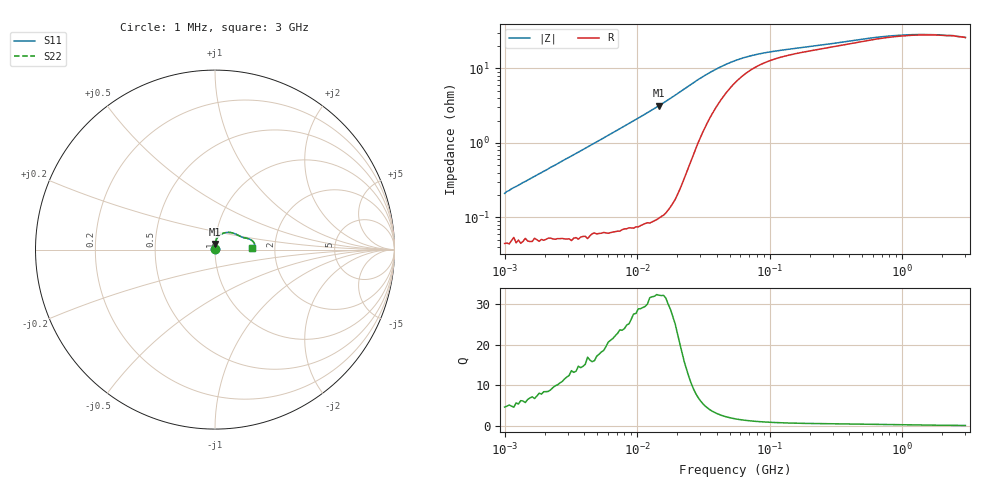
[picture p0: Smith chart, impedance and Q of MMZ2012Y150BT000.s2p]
! S-parameter Generated by TDK Corporation
! Copyright(C) 2016 TDK Corporation.
! All Rights Reserved.
! TDK P/N: MMZ2012Y150BT000 (Chip Beads)
! Property: |Z|=15¶ at 100MHz
! Size(LxWxT): 2x1.25x0.85mm, 0.079x0.049x0.033inches
! Model Type: s2p (Touchstone File Format Version 1.0)
! Frequency: DC=Yes Start=1MHz Stop=3000MHz 202points Log-sweep
! Note: This model was converted from impedance.
! Model Generated on May. 16, 2016
! Hash(MD5):
! Port Assignments:
!  1 ---@@@--- 2
! Applicable Conditions:
!  Temperature = 25 degC
!  DC Bias Current = 0 A
!  Small Signal Operation
! Terms and conditions regarding TDK Simulation Models
! (1)This simulation model is being provided solely for informational purposes. Please refer to the specifications of the products in terms of detailed characteristics of such products.
! (2)In no event shall TDK Corporation of any of its subsidiaries be liable for any loss or damage arising, directly or indirectly,
!  From any information contained in this simulation model, including, but not limited to loss or damages arising from any inaccuracies, omissions or errors in connection with such information.
! (3)Any and all copyrights on this simulation model are owned by TDK Corporation.
!  Duplication or redistribution of this simulation model without prior written permission from TDK Corporation is prohibited.
! (4)This simulation model is subject to any modification or change without any prior notice.
! (5)Neither TDK Corporation nor any of its subsidiaries shall make any warranty, express or implied,
!  Including but not limited to the correctness, implied warranties of merchantability and fitness for a particular purpose with respect to this simulation models.
! (6)The use of this simulation model shall be deemed to have consented to the terms and conditions hereof.
# MHz S MA R 50
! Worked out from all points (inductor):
!   201 points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, 1 MHz to 3 GHz, reference 50 ohm
!   read as one part in series: L = 33.4 nH near 1.041 MHz
!   highest Q = 32.1 at 14.62 MHz (marker M1), where L = 34.4 nH
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1  0.002106 77.6  0.9996 -0.1  0.9996 -0.1  0.002106 77.6
1.040844  0.002237 78.2  0.9995 -0.1  0.9995 -0.1  0.002237 78.2
1.083356  0.0023 78.8  0.9996 -0.1  0.9996 -0.1  0.0023 78.8
1.127605  0.002426 78.2  0.9995 -0.1  0.9995 -0.1  0.002426 78.2
2.055611  0.004312 83.0  0.9995 -0.2  0.9995 -0.2  0.004312 83.0
2.226959  0.004714 83.3  0.9995 -0.3  0.9995 -0.3  0.004714 83.3
3.900413  0.008162 85.6  0.9994 -0.5  0.9994 -0.5  0.008162 85.6
7.703107  0.01616 86.6  0.9992 -0.9  0.9992 -0.9  0.01616 86.6
14.61624  0.0316 86.4  0.9985 -1.8  0.9985 -1.8  0.0316 86.4
23.62996  0.05553 82.7  0.9945 -3.2  0.9945 -3.2  0.05553 82.7
32.54976  0.07933 74.0  0.9811 -4.5  0.9811 -4.5  0.07933 74.0
43.07715  0.1016 63.4  0.9588 -5.4  0.9588 -5.4  0.1016 63.4
54.77226  0.1189 53.8  0.9347 -5.9  0.9347 -5.9  0.1189 53.8
69.64249  0.1327 45.0  0.9111 -5.9  0.9111 -5.9  0.1327 45.0
88.54986  0.1429 37.9  0.8915 -5.6  0.8915 -5.6  0.1429 37.9
213.6344  0.1689 23.7  0.8481 -4.6  0.8481 -4.6  0.1689 23.7
536.4635  0.2031 16.3  0.8072 -4.1  0.8072 -4.1  0.2031 16.3
800.5644  0.2155 12.5  0.7909 -3.4  0.7909 -3.4  0.2155 12.5
1147.801  0.2218 9.1  0.7818 -2.6  0.7818 -2.6  0.2218 9.1
1645.649  0.222 6.2  0.7797 -1.8  0.7797 -1.8  0.222 6.2
2455.801  0.2161 3.8  0.7845 -1.0  0.7845 -1.0  0.2161 3.8
3000  0.2068 2.9  0.7936 -0.8  0.7936 -0.8  0.2068 2.9
